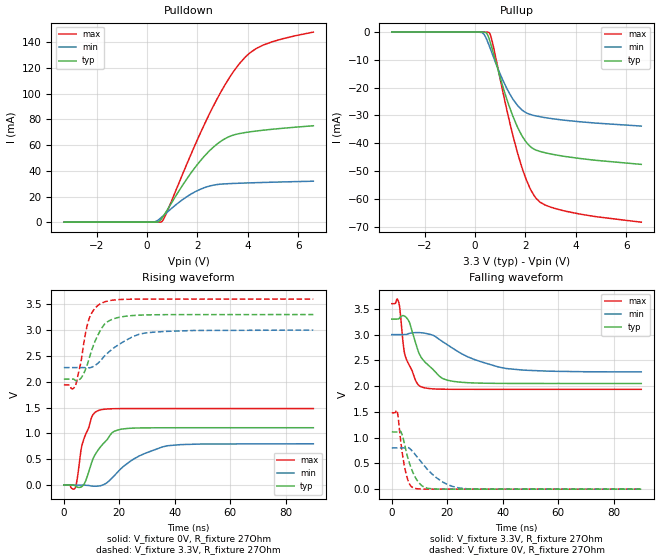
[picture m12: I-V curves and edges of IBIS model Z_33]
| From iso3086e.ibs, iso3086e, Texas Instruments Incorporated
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|   Z_33 Model
[Model]   Z_33
Model_type   3-state
|Signals   Z   negative pin
Polarity   Non-Inverting
Enable   Active-Low
Vmeas   = 1.57
Vref   = 1.65
Cref   = 50pF
|Rref = 27   |Note: 54 Ohm differential load;
| C_comp   obtained at 20MHz
|   typ   min   max
C_comp   99.04fF   99.46fF   109.8fF
[Voltage Range]   3.3   3   3.6
[Temperature Range]   40   125   -40
[Pullup Reference]   3.3   3   3.6
[Pulldown Reference]   0   0   0
[Power Clamp Reference]   3.3   3   3.6
[GND Clamp Reference]   0   0   0
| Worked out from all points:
|   slope of the pulldown table from 0 to 0.495 V, typ, clamps not added: 570 ohm
|   slope of the pullup table from 0 to 0.495 V, typ, clamps not added: 541 ohm
|   falling waveform, V_fixture 3.3V, R_fixture 27Ohm: 20-80 % time 7.84ns typ, 16.9ns min, 4.18ns max; typ from 3.3 V to 2.05 V
|   rising waveform, V_fixture 0V, R_fixture 27Ohm: 20-80 % time 6.95ns typ, 12.7ns min, 4.07ns max; typ from 0 V to 1.11 V
|   rising waveform, V_fixture 3.3V, R_fixture 27Ohm: 20-80 % time 5.57ns typ, 10.8ns min, 3.76ns max; typ from 2.05 V to 3.3 V
|   falling waveform, V_fixture 0V, R_fixture 27Ohm: 20-80 % time 4.01ns typ, 8.81ns min, 2.46ns max; typ from 1.11 V to 0 V
[Pulldown]
|   Voltage   I(typ)   I(min)   I(max)
-3.3V     -18.85fA   -97.11fA   -6.182fA
278.8mV   1.271uA    144.4uA    93.6nA
457.1mV   367.1uA    1.907mA    2.084uA
585.7mV   2.907mA    4.012mA    473.4uA
778.8mV   8.769mA    7.395mA    7.406mA
1.457V    30.15mA    18.22mA    39.56mA
2.289V    51.71mA    26.98mA    76.66mA
3.011V    64.08mA    29.76mA    104.2mA
3.645V    68.95mA    30.34mA    123mA
4.1V      70.43mA    30.65mA    132.2mA
4.59V     71.61mA    30.94mA    137.8mA
6.6V      75.12mA    31.93mA    148.1mA
[Pullup]
|   Voltage   I(typ)   I(min)   I(max)
-3.3V     225.7fA    -372fA     238.7fA
273.9mV   -1.35uA    -135.4uA   -350.5nA
447.1mV   -288uA     -2.26mA    -1.63uA
556.1mV   -2.246mA   -4.69mA    -159.8uA
694.6mV   -6.427mA   -8.027mA   -3.721mA
1.135V    -20.45mA   -17.86mA   -22.68mA
1.516V    -30.53mA   -24.28mA   -37.61mA
1.996V    -39.15mA   -28.85mA   -52.14mA
2.422V    -42.45mA   -30.17mA   -59.74mA
2.784V    -43.42mA   -30.78mA   -62.22mA
3.6V      -44.78mA   -31.76mA   -64.45mA
6.6V      -47.6mA    -33.82mA   -68.4mA
[Ramp]
R_load = 27
|   typ   min   max
dV/dt_r   0.66624/6.94669e-009  0.479874/1.27383e-008  0.888868/4.07021e-009
dV/dt_f   0.749267/7.85305e-009  0.434854/1.69152e-008  0.997391/4.19008e-009
[Falling Waveform]
V_fixture = 3.3V
V_fixture_min = 3V
V_fixture_max = 3.6V
R_fixture = 27Ohm
C_fixture = 0F
|   Time   V(typ)   V(min)   V(max)
0s        3.3V       3V         3.6V
2.32ns    3.304V     3V         3.658V
2.84ns    3.328V     3V         3.53V
4.8ns     3.351V     3.002V     2.593V
6.36ns    3.238V     3.025V     2.398V
8.88ns    2.785V     3.039V     2.078V
10.88ns   2.535V     3.035V     1.981V
19.72ns   2.119V     2.814V     1.939V
41.16ns   2.053V     2.342V     1.938V
89.92ns   2.051V     2.275V     1.938V
[Rising Waveform]
|Vcc
V_fixture = 0V
V_fixture_min = 0V
V_fixture_max = 0V
R_fixture = 27Ohm
C_fixture = 0F
|   Time   V(typ)   V(min)   V(max)
0s        3.791nV    141.5nV    3.857nV
4.12ns    -13.01mV   -3.914uV   -48.27mV
6.2ns     -36.46mV   138.7uV    687.1mV
6.96ns    -2.745mV   547.2uV    852.1mV
10.28ns   477.9mV    -19.69mV   1.344V
12.8ns    713mV      -15.58mV   1.45V
20ns      1.074V     287.2mV    1.48V
27.28ns   1.106V     567.4mV    1.481V
37.24ns   1.11V      760.8mV    1.481V
89.92ns   1.11V      799.8mV    1.481V
[Rising Waveform]
V_fixture = 3.3V
V_fixture_min = 3V
V_fixture_max = 3.6V
R_fixture = 27Ohm
C_fixture = 0F
|   Time   V(typ)   V(min)   V(max)
0s        2.051V     2.274V     1.938V
4.04ns    2.033V     2.274V     1.911V
6.64ns    2.107V     2.275V     2.55V
7.84ns    2.245V     2.269V     2.949V
9.12ns    2.452V     2.271V     3.224V
11.48ns   2.813V     2.324V     3.437V
14.68ns   3.115V     2.5V       3.545V
19.6ns    3.243V     2.713V     3.589V
29.16ns   3.292V     2.942V     3.599V
89.92ns   3.3V       3V         3.6V
[Falling Waveform]
|Gnd
V_fixture = 0V
V_fixture_min = 0V
V_fixture_max = 0V
R_fixture = 27Ohm
C_fixture = 0F
|   Time   V(typ)   V(min)   V(max)
0s        1.111V     800.5mV    1.482V
1.92ns    1.111V     800.5mV    1.511V
3.28ns    1.113V     800.4mV    900.6mV
4.96ns    787.3mV    802.6mV    342.7mV
6.36ns    504.1mV    793.8mV    101.4mV
8.12ns    265.3mV    692mV      18.96mV
12.76ns   18.5mV     388.6mV    432.9uV
17.96ns   1.449mV    150.8mV    157.2uV
24.36ns   34.45uV    22.14mV    128.8uV
89.92ns   56.36uV    77.77uV    40.93uV
